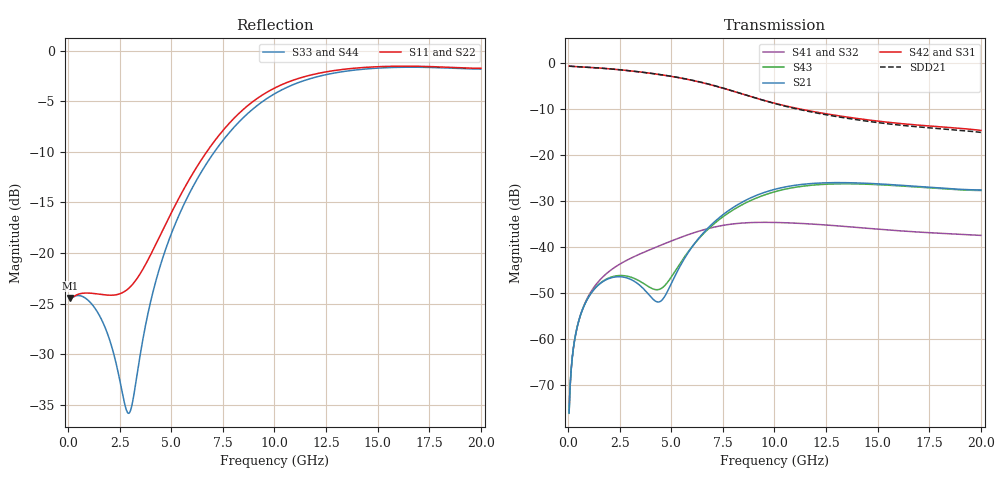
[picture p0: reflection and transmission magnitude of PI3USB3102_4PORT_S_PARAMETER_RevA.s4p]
! NPort=4 DATA=800 NOISE=0 GROUPDELAY=0 COMPLEX_DATAFORMAT=POLAR
! NumOfBlock=1 NumOfParam=0
! .MODEL Smodel S TSTONEFILE=PI3USB3102_4PORT_S_PARAMETER_RevA.s4p TYPE=S
!  -- The above .MODEL line can be used for the S element in the netlist.
! PORT DEFINITION
! PORT1 = INPUT+
! PORT2 = INPUT-
! PORT3 = OUTPUT+
! PORT4 = OUTPUT-
# Hz S MA R  50
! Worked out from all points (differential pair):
!   800 points, 50 MHz to 20 GHz, reference 50 ohm
!   strongest paths, dB at 50 MHz, 5.044 GHz, 10.04 GHz, 15.03 GHz, 20 GHz:
!     S42: -0.6, -2.9, -8.7, -12.6, -14.6
!     S31: -0.6, -2.9, -8.7, -12.6, -14.6
!     S21: -76.1, -47.5, -27.4, -26.2, -27.6
!     S43: -76.1, -46.2, -27.9, -26.4, -27.7
!     S41: -76.2, -38.6, -34.6, -36.1, -37.5
!     S32: -76.2, -38.6, -34.6, -36.1, -37.5
!   taken as a pair (ports 2,1 in; 4,3 out), SDD21 dB: -0.6, -2.8, -8.8, -12.9, -15.0
!   lowest |S11| = -24.5 dB at 99.94 MHz (marker M1), VSWR 1.13, Z = 56.3 - j0.594 ohm
!   |S11| at or under -10 dB: start of sweep to 6.713 GHz
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5e7  0.06037 -3.4  0.0001565 88.8  0.932 -1.1  0.0001552 88.7
     0.0001565 88.8  0.06037 -3.4  0.0001552 88.7  0.932 -1.1
     0.932 -1.1  0.0001552 88.7  0.06043 -2.5  0.0001565 88.8
     0.0001552 88.7  0.932 -1.1  0.0001565 88.8  0.06043 -2.5
9.99374e7  0.05984 -5.0  0.000312 87.8  0.9304 -2.2  0.0003095 87.6
           0.000312 87.8  0.05984 -5.0  0.0003095 87.6  0.9304 -2.2
           0.9304 -2.2  0.0003095 87.6  0.05988 -3.2  0.000312 87.9
           0.0003095 87.6  0.9304 -2.2  0.000312 87.9  0.05988 -3.2
9.23905e8  0.06336 -46.8  0.002687 72.2  0.907 -17.3  0.002758 70.6
           0.002687 72.2  0.06336 -46.8  0.002758 70.6  0.907 -17.3
           0.9071 -17.3  0.002758 70.6  0.05888 -30.9  0.002695 73.4
           0.002758 70.6  0.9071 -17.3  0.002695 73.4  0.05888 -30.9
2.94637e9  0.06698 -165.1  0.004539 44.5  0.8321 -52.8  0.007393 36.6
           0.004539 44.5  0.06698 -165.1  0.007393 36.6  0.8321 -52.8
           0.8321 -52.8  0.007393 36.6  0.0161 -167.5  0.004778 49.3
           0.007393 36.6  0.8321 -52.8  0.004778 49.3  0.0161 -167.5
5.49318e9  0.1972 77.9  0.006604 130.6  0.6895 -95.9  0.01285 2.9
           0.006604 130.6  0.1972 77.9  0.01285 2.9  0.6895 -95.9
           0.6896 -95.8  0.01285 2.9  0.1638 55.3  0.007002 118.8
           0.01285 2.9  0.6896 -95.8  0.007002 118.8  0.1638 55.3
1.02123e10  0.6706 -25.5  0.04367 72.0  0.3584 -158.7  0.0185 -79.3
            0.04367 72.0  0.6706 -25.5  0.0185 -79.3  0.3584 -158.7
            0.3585 -158.6  0.01851 -79.2  0.6305 -28.5  0.04116 70.7
            0.01851 -79.2  0.3585 -158.6  0.04116 70.7  0.6305 -28.5
2e10  0.8203 -102.4  0.04186 0.1  0.1861 100.1  0.0134 145.9
      0.04186 0.1  0.8203 -102.4  0.0134 145.9  0.1861 100.1
      0.1863 100.2  0.01341 145.9  0.813 -102.6  0.04135 0.5
      0.01341 145.9  0.1863 100.2  0.04135 0.5  0.813 -102.6
